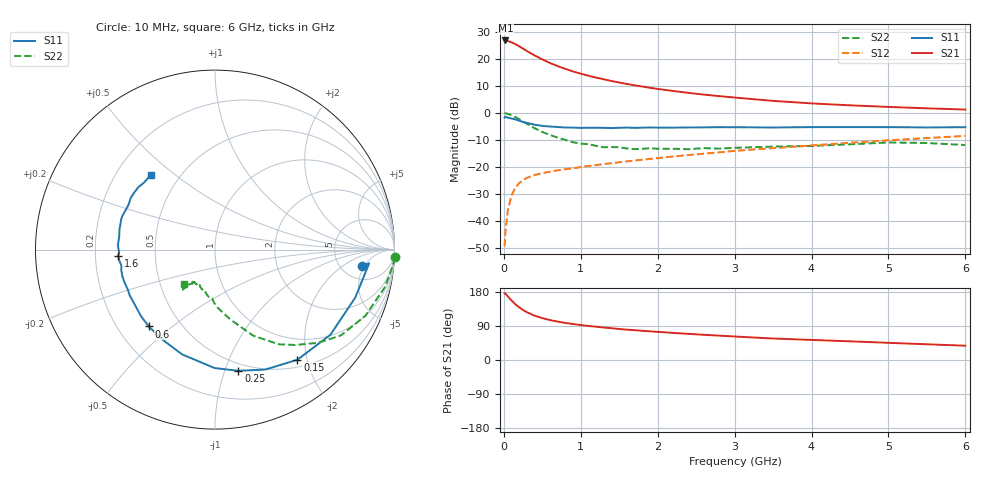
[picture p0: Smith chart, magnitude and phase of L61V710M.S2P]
!  INFINEON TECHNOLOGIES Small Signal Semiconductors
! BFR380L3 , Si-NPN RF-Transistor in TSLP-3-1
!  Vce=1.75 V,  Ic=10 mA
! Common Emitter S-Parameters:  07. March 2005
#  GHz  S  MA  R  50
! f  S11  S21  S12  S22
! GHz  Mag  Ang  Mag  Ang  Mag  Ang  Mag  Ang
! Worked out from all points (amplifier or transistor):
!   36 points, 10 MHz to 6 GHz, reference 50 ohm
!   highest |S21| = 27.0 dB at 20 MHz (marker M1)
!   |S21| within 3 dB of that: start of sweep to 247.7 MHz
!   unconditionally stable (mu >= 1): 2.178 GHz to 4.839 GHz
!   at 250 MHz: K = 0.26, MSG = 24.4 dB, |S12| = -24.9 dB
!   at 1.4 GHz: K = 0.88, MSG = 15.3 dB, |S12| = -18.6 dB
!   at 6 GHz: K = 0.97, MSG = 4.9 dB, |S12| = -8.4 dB
!   S11 on the Smith chart (normalised r, x): 10 MHz: 7.88, -4.47; 150 MHz: 0.62, -1.83; 250 MHz: 0.43, -1.11; 600 MHz: 0.33, -0.42; 1.6 GHz: 0.30, -0.03; 6 GHz: 0.35, +0.41
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0.01  0.8253 -6.3  22.33 175.8  0.0034 82.5  1.005 -2.5
0.02  0.8624 -5.1  22.38 175.3  0.0062 92.0  0.9942 -5.2
0.05  0.8258 -18.9  21.87 168.1  0.0153 79.5  0.9704 -12.3
0.1  0.799 -36.5  20.66 157.1  0.0297 74.0  0.9153 -23.8
0.15  0.7663 -53.2  19.15 147.1  0.0417 65.1  0.8489 -34.3
0.2  0.7249 -67.2  17.39 138.7  0.0505 60.1  0.7734 -42.2
0.25  0.6876 -79.1  15.77 132.0  0.0572 55.4  0.6948 -49.9
0.3  0.66 -90.2  14.23 126.0  0.0631 52.3  0.6365 -56.0
0.4  0.6119 -107.4  11.8 117.0  0.0712 48.1  0.5254 -66.0
0.5  0.5808 -120.3  9.963 110.6  0.0772 46.4  0.4484 -72.1
0.6  0.5651 -130.7  8.528 105.3  0.0818 45.9  0.3943 -78.0
0.7  0.5543 -138.2  7.477 101.3  0.0869 45.9  0.3507 -83.3
0.8  0.542 -145.5  6.64 97.8  0.0912 46.5  0.3188 -88.2
0.9  0.5394 -151.7  5.947 94.9  0.0945 47.1  0.2886 -91.8
1.1  0.5361 -160.0  4.958 89.8  0.1047 49.0  0.2654 -97.8
1.4  0.5291 -170.1  3.953 83.9  0.1175 51.1  0.2351 -104.8
1.6  0.5406 -176.4  3.486 80.1  0.1274 52.4  0.2207 -112.5
2.2  0.5388 171.8  2.585 71.5  0.1571 56.0  0.2186 -117.7
3.5  0.5427 152.5  1.691 56.7  0.2242 58.4  0.2395 -126.4
4.5  0.551 145.3  1.399 49.3  0.2824 59.1  0.2643 -128.0
5.5  0.5437 136.3  1.23 41.5  0.3455 57.0  0.2793 -129.5
6  0.5495 130.7  1.168 37.7  0.3786 55.4  0.2563 -131.8
